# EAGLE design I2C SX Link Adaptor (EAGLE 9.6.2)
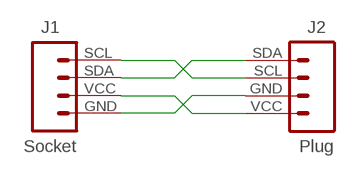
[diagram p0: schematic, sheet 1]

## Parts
J1  Socket  HEADER-1X4-I2C-SX  [CONN_04-I2C-SX]
J2  Plug  HEADER-1X4-I2C  [CONN_04-I2C]

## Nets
N$1: J1.SDA J2.SDA
N$2: J1.SCL J2.SCL
N$3: J1.GND J2.GND
N$5: J1.VCC J2.VCC

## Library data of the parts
J1 = digitalconcepts:HEADER-1X4-I2C-SX: I2C Interface [Pin 1 GND & Pin 3 SDA] 4-Pin Header
J2 = digitalconcepts:HEADER-1X4-I2C: I2C Interface [Pin 1 Vcc] 4-Pin Header

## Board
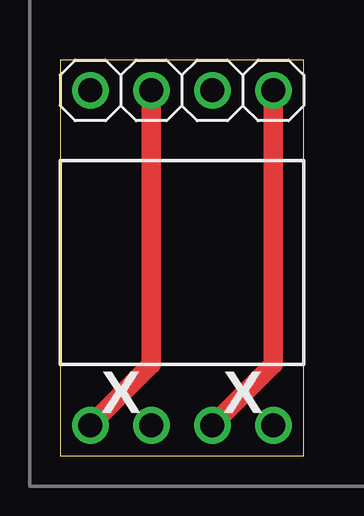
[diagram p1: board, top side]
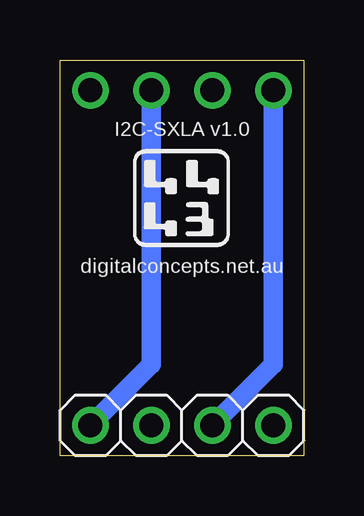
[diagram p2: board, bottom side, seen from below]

Size 10.16 x 16.51 mm. Coordinates in mm from the lower left corner, seen from the top.
Outline: 0,0 10.16,0 10.16,16.51 0,16.51 0,0
Copper layers (1*16): Top 0.035mm / dielectric 1.5mm / Bottom 0.035mm
Design rules "default *": minimum track width 6mil, minimum drill 0.35mm, track to track 6mil, track to pad 6mil, pad to pad 6mil, via to via 6mil, smd to smd 6mil, copper to edge 15mil, drill to drill 6mil, minimum pad ring 10mil, minimum via ring 8mil, stop-mask expansion 4mil, vias tented up to drill 0mil, thermal gap 10mil

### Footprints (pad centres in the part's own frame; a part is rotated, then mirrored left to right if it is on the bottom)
CONN_04-I2C-SX = drill 1 pad 1.524: GND 0,0; SCL 7.62,0; SDA 5.08,0; VCC 2.54,0
CONN_04-I2C = drill 1 pad 1.524: GND 2.54,0; SCL 5.08,0; SDA 7.62,0; VCC 0,0

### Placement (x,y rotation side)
J1  1.27,1.27 180 bottom
J2  1.27,15.24 0 top

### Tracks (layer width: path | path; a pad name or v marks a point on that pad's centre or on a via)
N$1
  Top 0.813: J1.SDA 8.89,3.81 J2.SDA
N$2
  Bottom 0.813: J2.SCL 6.35,3.81 J1.SCL
N$3
  Top 0.813: J2.GND 3.81,3.81 J1.GND
N$5
  Bottom 0.813: J2.VCC 1.27,3.81 J1.VCC

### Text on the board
tPlace: X | X
bPlace: I2C-SXLA v1.0 | digitalconcepts.net.au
